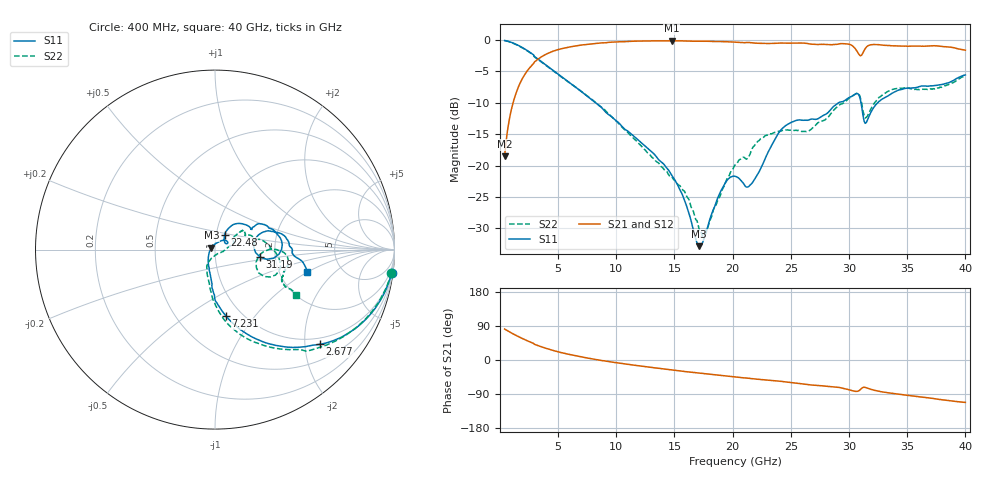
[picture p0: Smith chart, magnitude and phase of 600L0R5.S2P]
!  American Technical Ceramics  Date:  10/27/06
!  One Norden Lane
!  Huntington Station,  NY.  11746-2102
!  Tel:  (631) 622-4700  Fax:  (631) 622-4748
!  Part Number  600L0R5
!  Description: Ultra Low ESR Microwave capacitors
!  Application: Coupling, Bypass, Tuning, DC Block
!  Filters, Matching
# GHZ S DB R 50
! Freq  |S11|  S11 Ph  |S21|  S21 Ph  |S12|  S12 Ph  |S22|  S22 Ph
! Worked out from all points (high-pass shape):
!   401 points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, 400 MHz to 40 GHz, reference 50 ohm
!   highest |S21| = -0.11 dB at 14.76 GHz (marker M1); lowest = -18.5 dB at 400 MHz (marker M2)
!   |S21| within 3 dB of the highest: 3.225 GHz to end of sweep
!   lowest |S11| = -32.8 dB at 17.13 GHz (marker M3), VSWR 1.05, Z = 48 + j0.956 ohm
!   |S11| at or under -10 dB: 8.221 GHz to 29.09 GHz (20.87 GHz wide, 112 % of centre); 31.03 GHz to 32.45 GHz (1.423 GHz wide, 4.48 % of centre)
!   |S22| runs from -31.4 to -0.1 dB; largest |S21 - S12| = 0.0035
!   S11 on the Smith chart (normalised r, x): 400 MHz: 1, -15; 2.677 GHz: 0.84, -2.34; 7.231 GHz: 0.84, -0.72; 22.48 GHz: 1.10, +0.18; 31.19 GHz: 1.66, -0.15; 40 GHz: 2.85, -0.99
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0.4  -0.06 -7.7  -18.49 81.7  -18.48 81.7  -0.09 -7.5
1.291  -0.60 -23.4  -8.96 66.3  -8.96 66.2  -0.62 -23.3
2.677  -2.08 -42.1  -4.15 46.6  -4.16 46.5  -2.12 -45.0
4.558  -4.82 -62.9  -1.77 25.3  -1.78 25.3  -4.88 -65.8
7.033  -8.26 -79.6  -0.78 7.9  -0.78 7.9  -8.23 -83.1
7.231  -8.54 -80.7  -0.73 6.8  -0.73 6.8  -8.50 -84.0
13.666  -19.11 -106.8  -0.12 -22.1  -0.12 -22.1  -19.66 -116.4
14.755  -21.50 -116.2  -0.11 -26.2  -0.11 -26.2  -21.72 -117.5
17.131  -32.84 154.1  -0.19 -34.5  -0.19 -34.6  -30.25 -86.8
17.626  -31.06 100.2  -0.18 -36.2  -0.18 -36.2  -30.63 -47.1
19.012  -23.95 52.5  -0.24 -40.9  -0.25 -40.9  -24.30 2.9
20.2  -21.70 30.5  -0.32 -44.8  -0.32 -44.9  -19.90 17.1
21.289  -23.42 35.8  -0.39 -48.0  -0.38 -48.1  -18.81 27.4
22.477  -20.22 56.7  -0.52 -51.6  -0.52 -51.7  -15.67 34.6
24.358  -13.93 46.3  -0.48 -57.2  -0.48 -57.3  -14.38 33.7
26.833  -12.58 28.7  -0.66 -66.1  -0.66 -66.2  -14.06 24.7
29.902  -9.27 18.5  -0.63 -77.4  -0.64 -77.5  -9.42 -2.6
30.595  -8.54 7.5  -1.53 -82.8  -1.53 -82.9  -8.54 -12.7
31.189  -11.87 -9.5  -2.06 -72.5  -2.07 -72.6  -11.18 -28.1
31.981  -11.15 19.8  -0.72 -78.3  -0.72 -78.5  -10.65 -0.5
33.466  -8.75 14.8  -0.87 -86.9  -0.88 -87.0  -8.07 -3.9
40  -5.56 -13.7  -1.61 -111.9  -1.62 -112.1  -5.72 -29.5
